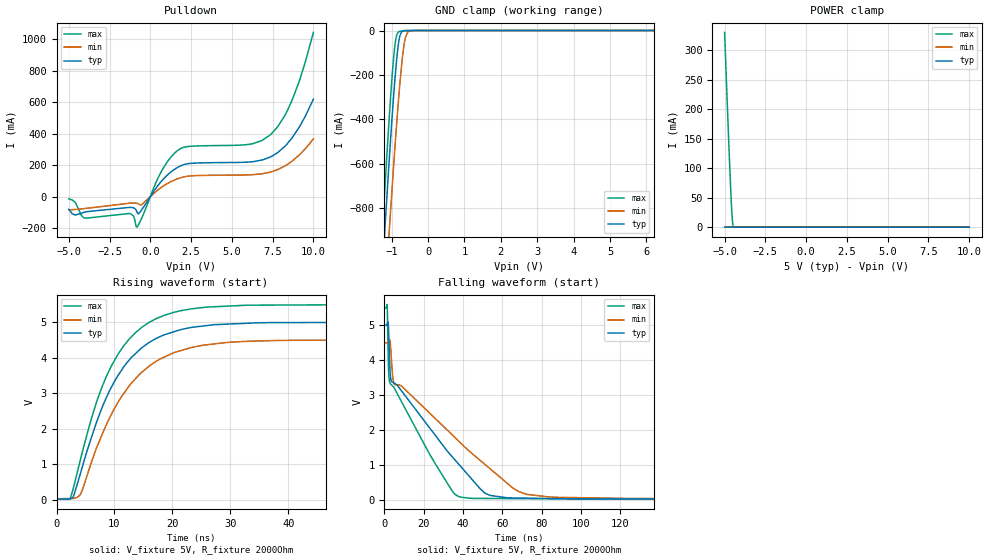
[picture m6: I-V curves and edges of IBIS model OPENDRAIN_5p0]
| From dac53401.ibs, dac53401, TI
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|   OPENDRAIN_5p0 Model
[Model]   OPENDRAIN_5p0
Model_type   I/O_open_drain
Polarity   Non-Inverting
Enable   Active-Low
Vinl = 0.4
Vinh = 1.62
Vmeas = 2.5
Vref = 5
Cref = 2pF
Rref = 2000
|   typ   min   max
C_comp   1.041pF   1.018pF   1.056pF
[Voltage Range]   5   4.5   5.5
[Temperature Range]   25   125   -40
[Pullup Reference]   5   4.5   5.5
[Pulldown Reference]   -0   -0   0
[Power Clamp Reference]   5   4.5   5.5
[GND Clamp Reference]   0   0   0
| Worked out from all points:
|   slope of the pulldown table from 0 to 0.75 V, typ, clamps not added: 7.08 ohm
|   GND clamp passes 1 mA (typ) near -0.66 V on its own axis
|   falling waveform, V_fixture 5V, R_fixture 2000Ohm: 20-80 % time 35.2ns typ, 49ns min, 23.2ns max; typ from 5 V to 0.015 V
|   rising waveform, V_fixture 5V, R_fixture 2000Ohm: 20-80 % time 8.29ns typ, 9.08ns min, 7.85ns max; typ from 0.015 V to 5 V
[Pulldown]
|   Voltage   I(typ)   I(min)   I(max)
-5V       -80.51mA   -84.93mA   -14.22mA
-4.61V    -116.6mA   -81.76mA   -36.26mA
-4.055V   -99.11mA   -76.39mA   -136.3mA
-1.25V    -68.27mA   -41.68mA   -106.9mA
-815mV    -98.03mA   -42.8mA    -193.3mA
-545mV    -86.42mA   -51.89mA   -140.3mA
640mV     92.99mA    55.98mA    152.9mA
1.69V     186.9mA    114.2mA    294.7mA
6.115V    220.5mA    138.6mA    333.3mA
7.405V    254mA      157.2mA    397.4mA
8.68V     372mA      224.5mA    609.6mA
10V       619.9mA    367mA      1.044A
[GND Clamp]
|   Voltage   I(typ)   I(min)   I(max)
-5V       -11.57A    -11.14A    -12.21A
-1.25V    -1.062A    -1.374A    -881.6mA
-1.145V   -781.1mA   -1.101A    -592.5mA
-1.07V    -587.2mA   -910.3mA   -396.2mA
-980mV    -368.2mA   -688.1mA   -186.4mA
-920mV    -236.6mA   -546.1mA   -78.11mA
-860mV    -123.7mA   -411.3mA   -19.48mA
-785mV    -31mA      -257mA     -4.18mA
-710mV    -3.686mA   -127.3mA   -1.659mA
-650mV    -701.8uA   -53.65mA   -668.9uA
-515mV    -32.95uA   -2.223mA   -35.21uA
10V       0A         0A         0A
[POWER Clamp]
|   Voltage   I(typ)   I(min)   I(max)
-5V       960nA      3.539nA    330.6mA
-4.865V   0A         0A         231mA
-4.76V    0A         0A         155.3mA
-4.67V    0A         0A         93.19mA
-4.61V    0A         0A         54.75mA
-4.565V   0A         0A         29.41mA
-4.535V   0A         0A         15.78mA
-4.52V    0A         0A         10.49mA
-4.49V    0A         0A         3.647mA
-4.445V   0A         0A         475.5uA
10V       0A         0A         0A
[Ramp]
R_load = 2000
|   typ   min   max
dV/dt_r   2.99117/8.3009e-09   2.68662/9.05727e-09   3.29428/7.85179e-09
dV/dt_f   2.99117/3.50324e-08   2.68662/4.86741e-08   3.29428/2.31908e-08
[Falling Waveform]
V_fixture = 5V
V_fixture_min = 4.5V
V_fixture_max = 5.5V
R_fixture = 2000Ohm
C_fixture = 0F
|   Time   V(typ)   V(min)   V(max)
0s        5V         4.5V       5.5V
1.387ns   5.043V     4.501V     5.585V
2.1ns     4.854V     4.557V     3.728V
2.885ns   3.649V     4.525V     3.338V
5.106ns   3.337V     3.305V     3.189V
34.18ns   1.248V     1.874V     270.8mV
42.99ns   679.5mV    1.397V     42.9mV
68.41ns   44.68mV    230.2mV    30.29mV
87.6ns    29.31mV    66.99mV    25.05mV
1.5us     14.72mV    22.29mV    9.53mV
[Rising Waveform]
V_fixture = 5V
V_fixture_min = 4.5V
V_fixture_max = 5.5V
R_fixture = 2000Ohm
C_fixture = 0F
|   Time   V(typ)   V(min)   V(max)
0s        14.72mV    22.29mV    9.53mV
2.423ns   24.56mV    31.49mV    54.26mV
4.07ns    708.2mV    134.5mV    1.092V
5.834ns   1.659V     962.2mV    2.181V
8.301ns   2.765V     2.002V     3.356V
10.66ns   3.51V      2.757V     4.11V
13.6ns    4.111V     3.404V     4.703V
20.24ns   4.731V     4.142V     5.278V
32.93ns   4.971V     4.462V     5.481V
1.5us     5V         4.5V       5.5V
